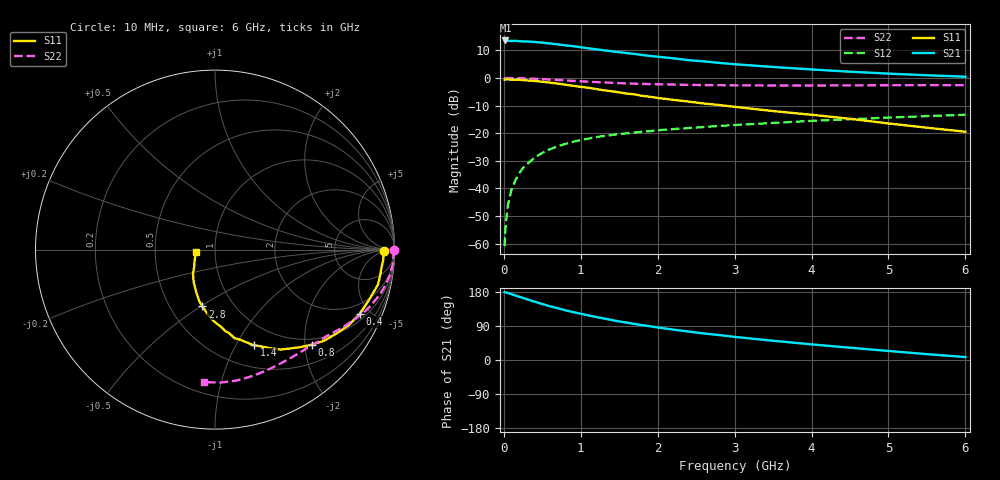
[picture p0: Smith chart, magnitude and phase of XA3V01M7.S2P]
! SIEMENS Discrete & RF Semiconductors
! BFY180
! Si NPN RF Bipolar Junction Transistor in MICRO-X
! VCE = 3 V  IC = 1.7 mA
! Common Emitter S-Parameters:  May  1997
# GHz  S  MA  R  50
!  f  S11  S21  S12  S22
! GHz  MAG  ANG  MAG  ANG  MAG  ANG  MAG  ANG
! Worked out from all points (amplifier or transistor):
!   36 points, 10 MHz to 6 GHz, reference 50 ohm
!   highest |S21| = 13.6 dB at 20 MHz (marker M1)
!   |S21| within 3 dB of that: start of sweep to 1.143 GHz
!   unconditionally stable (mu >= 1): 2.976 GHz to end of sweep
!   at 250 MHz: K = 0.10, MSG = 22.9 dB, |S12| = -32.5 dB
!   at 1.4 GHz: K = 0.64, MSG = 15.2 dB, |S12| = -20.7 dB
!   at 6 GHz: K = 1.07, MAG = 5.3 dB, |S12| = -13.3 dB
!   S11 on the Smith chart (normalised r, x): 10 MHz: 32, -5; 400 MHz: 1.34, -4.33; 800 MHz: 0.87, -2.15; 1.4 GHz: 0.75, -1.19; 2.8 GHz: 0.72, -0.51; 6 GHz: 0.81, -0.02
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0.01  0.9403 -0.5  4.696 179.2  0.0009 91.3  0.9963 -0.2
0.02  0.9373 -1.2  4.783 178.4  0.0018 98.9  0.9999 -0.6
0.05  0.9402 -3.2  4.716 176.8  0.0048 88.2  0.9963 -1.6
0.1  0.9339 -5.8  4.694 173.6  0.0096 86.0  0.9926 -3.2
0.15  0.9307 -9.4  4.705 170.2  0.014 84.1  0.9941 -4.8
0.25  0.9139 -15.2  4.585 163.8  0.0236 81.2  0.9869 -7.9
0.3  0.9027 -18.1  4.594 160.2  0.0274 78.7  0.9803 -9.3
0.4  0.8827 -23.9  4.492 153.9  0.0361 74.8  0.9671 -12.3
0.6  0.8235 -34.5  4.219 141.6  0.0513 68.1  0.9367 -17.5
0.8  0.7554 -44.5  3.901 131.1  0.0641 62.1  0.9041 -22.3
0.9  0.7222 -48.8  3.77 126.5  0.0699 59.6  0.8861 -24.4
1.1  0.6656 -56.8  3.444 117.7  0.0801 55.5  0.8558 -28.1
1.4  0.5762 -67.7  3.044 105.5  0.0927 50.3  0.8186 -33.2
1.5  0.5487 -70.9  2.937 101.7  0.0965 48.8  0.808 -34.7
1.8  0.4737 -80.2  2.604 92.0  0.1061 45.8  0.7814 -39.0
2.2  0.4025 -90.4  2.273 80.2  0.1187 41.5  0.7601 -44.5
2.6  0.3454 -98.8  1.999 70.0  0.1294 38.6  0.7448 -49.6
2.8  0.3243 -102.6  1.876 65.8  0.1355 37.2  0.7405 -52.1
3.5  0.2517 -115.2  1.582 50.8  0.1536 32.3  0.7319 -60.8
4.5  0.1825 -132.3  1.299 32.4  0.1798 25.3  0.7347 -73.8
5.5  0.1258 -154.3  1.12 15.4  0.2044 17.7  0.7415 -87.7
6  0.1063 -171.9  1.055 7.7  0.2156 13.4  0.7407 -94.8
